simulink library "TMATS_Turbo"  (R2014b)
settings: Solver=ode45  StartTime=0.0  StopTime=10.0  RelTol=1e-3
libraries: Lib_Turbo_Ambient_TMATS x1, Lib_Turbo_Burner_TMATS x1, Lib_Turbo_Compressor_TMATS x1, Lib_Turbo_Duct_TMATS x1, Lib_Turbo_FlowPathChar_TMATS x1, Lib_Turbo_GearBox_TMATS x1, Lib_Turbo_HeatXchang_TMATS x1, Lib_Turbo_Inlet_TMATS x1, Lib_Turbo_Mixer_TMATS x1, Lib_Turbo_Nozzle_TMATS x1, Lib_Turbo_PGenerator_TMATS x1, Lib_Turbo_SFCCalc_TMATS x1

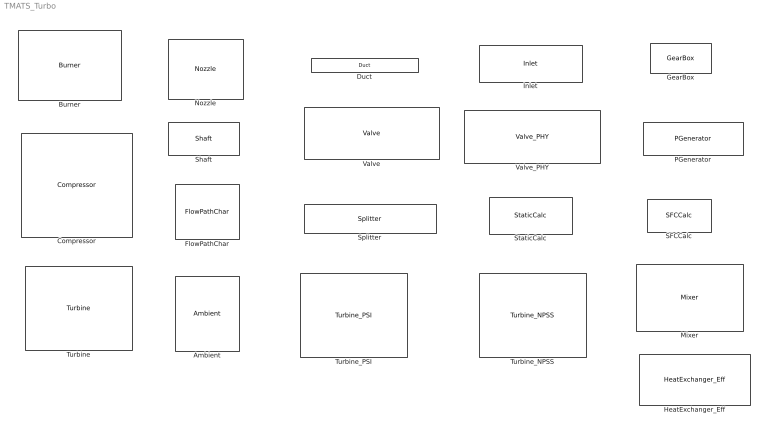
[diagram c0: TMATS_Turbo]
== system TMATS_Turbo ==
  Ambient : Lib_Turbo_Ambient_TMATS/Ambient  X_A_AltVec_M=5000*[-1 0 1 2 3 4 5 6 7 8 9 10 12 14 16]  T_A_TsVec_M=[536.51 518.67 500.84 483.03 465.22 447.41 429.62 411.84 394.06 389.97 389.97 389.97 389.97 392.25 397.69]  T_A_PsVec_M=[17.554 14.696 12.228 10.108 8.297 6.759 5.461 4.373 3.468 2.73 2.149 1.692 1.049 0.651 0.406]  AFARc_M=0  X_A_FARVec_M=[0; 0.0050; 0.0100; 0.0150; 0.0200; 0.0250; 0.0300]  T_A_RtArray_M="[0.0686;    0.0686;    0.0686;    0.0686;    0.0686;    0.0686;    0.0686]"  Y_A_TVec_M=[300 10000]  T_A_gammaArray_M=[ 1.4 1.4 1.4 1.4 1.4 1.4 1.4; 1.4 1.4 1.4 1.4 1.4 1.4 1.4]
  Burner : Lib_Turbo_Burner_TMATS/Burner  LHV_M=18400  dPnormBurner_M=0.05  Eff_M=1
  Compressor : Lib_Turbo_Compressor_TMATS/Compressor  X_C_RlineVec_M=[1.000 3.000 ]  Y_C_NcVec_M="[0.500  0.900  1.050]"  T_C_Map_WcArray_M=[0 0; 0 0; 0 0]  T_C_Map_PRArray_M=[0 0; 0 0; 0 0]  T_C_Map_EffArray_M=[0 0; 0 0; 0 0]  s_C_Nc_M=0.0001  s_C_Wc_M=0.4953  s_C_PR_M=0.8636  s_C_Eff_M=0.9977  CBLDEN_M=off  C_CBD_M=0  C_CBFht_M=0.5  C_CBFPt_M=0.5  FBLDEN_M=off  C_FBD_M=0  C_BFht_M=0.5  C_BFPt_M=0.5  X_C_WcSurgeVec_M=[0 200]  T_C_PRSurgeVec_M=[30 30]  iDesign_M=2  NcDes_M=10000  EffDes_M=0.95  PRDes_M=20  RlineDes_M=2  FVar_M='iDesScalars.mat'  SVar_M=gcb  NcNm_M='_C_Nc'  WcNm_M='_C_Wc'  PRNm_M='_C_PR'  EffNm_M='_C_Eff'
  Duct : Lib_Turbo_Duct_TMATS/Duct  dP_M=0.005
  FlowPathChar : Lib_Turbo_FlowPathChar_TMATS/FlowPathChar
  GearBox : Lib_Turbo_GearBox_TMATS/GearBox  R_M=2  Eff_M=.99
  HeatExchanger_Eff : Lib_Turbo_HeatXchang_TMATS/HeatExchanger_Eff  dP1_M=0.005  dP2_M=0.005  E_M=0.5  iDesign_M=2  dQDes_M=1000  FVar_M='iDesScalars.mat'  SVar_M=gcb  ENm_M='_E'
  Inlet : Lib_Turbo_Inlet_TMATS/Inlet  eRambase_M=1  X_eRamVec_M=[0 3]  T_eRamtbl_M=[1 1]
  Mixer : Lib_Turbo_Mixer_TMATS/Mixer  Aphy1_M=10  Aphy2_M=10  s_M_Imp1_M=1  s_M_Imp2_M=1  s_M_V1_M=1  s_M_V2_M=1  Y_M_FARVec_M=[0; 0.0050; 0.0100; 0.0150; 0.0200; 0.0250; 0.0300]  T_M_RtArray_M="[0.0686;    0.0686;    0.0686;    0.0686;    0.0686;    0.0686;    0.0686]"  X_M_TVec_M=[300 10000]  T_M_gammaArray_M=[ 1.4 1.4 1.4 1.4 1.4 1.4 1.4; 1.4 1.4 1.4 1.4 1.4 1.4 1.4]  iDesign_M=2  SWPS_M=0  BPRDes_M=0.5  MNDes_M=0.4  FVar_M='iDesScalars.mat'  SVar_M=gcb  Aphy1des_M='_Aphy1'  Aphy2des_M='_Aphy2'
  Nozzle : Lib_Turbo_Nozzle_TMATS/Nozzle  SWType_M=1  N_TArea_M=110.7  N_EArea_M=110.7  N_FL_M=0.00  X_N_TtVec2_M=[300 10000]  T_N_TGArray_M=[1 1]  X_N_PEQPaVec_M=[0 10000]  T_N_CdThArray_M=[1 1]  T_N_CvArray_M=[0.990 0.990]  T_N_CfgArray_M=[1 1]  X_N_FARVec_M=[0; 0.0050; 0.0100; 0.0150; 0.0200; 0.0250; 0.0300]  T_N_RtArray_M="[0.0686;    0.0686;    0.0686;    0.0686;    0.0686;    0.0686;    0.0686]"  Y_N_TtVec_M=[300 10000]  T_N_MAP_gammaArray_M=[ 1.4 1.4 1.4 1.4 1.4 1.4 1.4; 1.4 1.4 1.4 1.4 1.4 1.4 1.4]  iDesign_M=2  WDes_M=100  FVar_M='iDesScalars.mat'  SVar_M=gcb  AthNm_M='_Ath'  AxNm_M='_Ax'
  PGenerator : Lib_Turbo_PGenerator_TMATS/PGenerator  Eff_M=.995
  SFCCalc : Lib_Turbo_SFCCalc_TMATS/SFCCalc
  Shaft : Lib_Turbo_Shaft_TMATS/Shaft  Shaft_Inertia_M=0.3183
  Splitter : Lib_Turbo_Splitter_TMATS/Splitter
  StaticCalc : Lib_Turbo_StaticCalc_TMATS/StaticCalc  ST_M=off  Ath_M=100  MN_M=0.5  X_FARVec_M=[0; 0.0050; 0.0100; 0.0150; 0.0200; 0.0250; 0.0300]  Y_TtVec_M=[300 10000]  T_RtArray_M="[0.0686;    0.0686;    0.0686;    0.0686;    0.0686;    0.0686;    0.0686]"  T_gammaArray_M=[ 1.4 1.4 1.4 1.4 1.4 1.4 1.4; 1.4 1.4 1.4 1.4 1.4 1.4 1.4]
  Turbine : Lib_Turbo_Turbine_TMATS/Turbine  X_T_PRVec_M="[ 3.000  8.000]"  Y_T_NcVec_M="[60 80  110]"  T_T_Map_WcArray_M=[0 0;0 0; 0 0]  T_T_Map_EffArray_M=[0 0; 0 0; 0 0]  s_T_Nc_M=0.0243  s_T_Wc_M=0.4504  s_T_PR_M=0.9736  s_T_Eff_M=0.9984  CFlwEn_M=off  T_CoolFlwPos_M=0  iDesign_M=2  NcDes_M=100  EffDes_M=0.9328  PRDes_M=5  NDes_M=10000  FVar_M='iDesScalars.mat'  SVar_M=gcb  NcNm_M='_C_Nc'  WcNm_M='_C_Wc'  PRNm_M='_C_PR'  EffNm_M='_C_Eff'
  Turbine_NPSS : Lib_Turbo_TurbineNPSS_TMATS/Turbine_NPSS  X_T_PRVec_M="[ 3.000  8.000]"  Y_T_NcVec_M="[60 80  110]"  T_T_Map_WcArray_M=[0 0;0 0; 0 0]  T_T_Map_EffArray_M=[0 0; 0 0; 0 0]  s_T_Nc_M=0.0243  s_T_Wc_M=0.4504  s_T_PR_M=0.9736  s_T_Eff_M=0.9984  CFlwEn_M=off  T_CoolFlwPos_M=0  iDesign_M=2  NcDes_M=100  EffDes_M=0.9328  PRDes_M=5  NDes_M=10000  FVar_M='iDesScalars.mat'  SVar_M=gcb  NcNm_M='_C_Nc'  WcNm_M='_C_Wc'  PRNm_M='_C_PR'  EffNm_M='_C_Eff'
  Turbine_PSI : Lib_Turbo_TurbinePSI_TMATS/Turbine_PSI  X_T_PRpVec_M="[ 3.000  8.000]"  Y_T_NcpVec_M="[60 80  110]"  T_T_Map_PSIArray_M=[0 0; 0 0; 0 0]  X_T_PRwVec_M="[60 80  110]"  Y_T_NcwVec_M="[60 80  110]"  T_T_Map_WoWArray_M=[0 0;0 0; 0 0]  s_T_hi_M=0.1  s_T_Nc_M=0.0243  s_T_Wc_M=0.4504  s_T_PR_M=0.9736  s_T_Eff_M=0.9984  CFlwEn_M=off  T_CoolFlwPos_M=0  gamma_M=1.4  Rt_M=0.1  iDesign_M=2  NcDes_M=100  EffDes_M=0.9328  PRDes_M=5  NDes_M=10000  FVar_M='iDesScalars.mat'  SVar_M=gcb  NcNm_M='_C_Nc'  WcNm_M='_C_Wc'  PRNm_M='_C_PR'  EffNm_M='_C_Eff'
  Valve : Lib_Turbo_Valve_TMATS/Valve  VFO_M=1  VDZ_M=0  VAe_M=20  X_VPRVec_M=[1 10]  T_VWArray_M=[0 .99]
  Valve_PHY : Lib_Turbo_ValvePHY_TMATS/Valve_PHY  s_V_AeVLV_M=200  s_V_AeBYP_M=200  s_V_AeTH_M=167  X_V_FARVec_M=[0 1]  T_V_RtVec_M=[0 .99]  Y_V_TtVec_M=[1 10000]  T_V_gammaArray_M=[1.4 1.4; 1.4 1.4]
